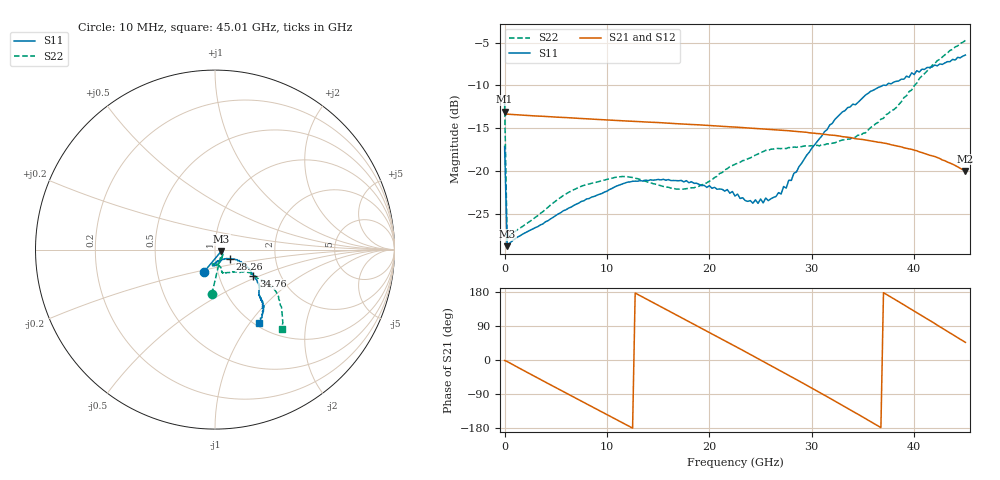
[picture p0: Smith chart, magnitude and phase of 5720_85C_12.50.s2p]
! Device:  ADRF5720
! Description: 0.5dB LSB GaAs MMIC 6-bit Digital Attenuator
! Frequency:  0.000009 -  40 GHz
! Ports:
!	RF1	= Port 1
!	RF2	= Port 2
! Vdd:  3.3 Volt
! Vss:  -3.3 Volt
! Control:  0/3.3 Volt
! State:  12.50 dB attenuation
! Data:  The device was measured using G-S-G Probes on a matrix board.
!  Data was collected using an calibrated 4 port network analyzer.
!  The reference plane for this measurement is at the launchers.
! Note:  Analog Devices supplies this data as a sample of measured data
!  for this product.  Your particular data for this product may vary.
!  Data was taken at 85 degrees C.
!  Analog Devices reserves the right to change this data at anytime.
# GHZ S DB R 45.0
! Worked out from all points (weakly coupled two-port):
!   181 points, 10 MHz to 45.01 GHz, reference 45 ohm
!   highest |S21| = -13.07 dB at 10 MHz (marker M1); lowest = -20.0 dB at 45.01 GHz (marker M2)
!   lowest |S11| = -28.8 dB at 260 MHz (marker M3), VSWR 1.08, Z = 48.3 - j0.813 ohm
!   |S11| at or under -10 dB: start of sweep to 36.96 GHz; 37.1975 GHz to 37.27 GHz (72.5 MHz wide, 0.195 % of centre)
!   |S22| runs from -28.0 to -4.8 dB; largest |S21 - S12| = 0.001
!   S11 on the Smith chart (normalised r, x): 10 MHz: 0.86, -0.22; 28.26 GHz: 1.17, -0.12; 34.76 GHz: 1.46, -0.46; 45.01 GHz: 1.05, -1.11
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0.01  -17.14 -116.3  -13.07 -1.3  -13.05 -1.3  -12.10 -94.1
0.26  -28.81 -13.4  -13.37 -4.0  -13.37 -4.0  -28.03 -12.8
2.26  -27.09 -15.1  -13.52 -33.4  -13.51 -33.3  -26.08 -25.4
4.26  -25.83 -36.9  -13.66 -62.1  -13.64 -62.1  -24.25 -52.7
7.76  -23.50 -59.0  -13.89 -112.1  -13.88 -112.1  -21.70 -78.5
11.51  -21.52 -78.4  -14.14 -165.5  -14.13 -165.4  -20.66 -95.9
15.26  -21.06 -91.3  -14.37 140.9  -14.36 141.0  -21.74 -99.5
19.01  -21.59 -94.5  -14.62 87.1  -14.61 87.3  -21.80 -82.1
22.76  -22.72 -84.2  -14.90 32.9  -14.89 33.1  -19.11 -72.0
24.26  -23.79 -74.9  -15.02 11.1  -15.01 11.3  -18.31 -72.1
25.01  -23.29 -67.4  -15.07 0.1  -15.06 0.3  -17.87 -73.1
25.26  -23.75 -66.1  -15.09 -3.5  -15.07 -3.3  -17.75 -72.5
25.51  -23.18 -61.7  -15.11 -7.2  -15.09 -7.0  -17.60 -73.2
27.01  -22.71 -43.9  -15.23 -29.4  -15.22 -29.1  -17.40 -71.5
28.26  -20.28 -31.4  -15.37 -48.0  -15.36 -47.7  -17.21 -71.5
30.26  -16.99 -26.2  -15.60 -78.0  -15.58 -77.7  -17.17 -68.0
33.01  -13.10 -29.4  -16.00 -120.0  -15.98 -119.8  -16.39 -57.6
34.76  -11.72 -34.3  -16.29 -146.9  -16.27 -146.6  -15.88 -50.2
37.76  -9.82 -40.7  -16.95 165.5  -16.93 165.9  -12.97 -34.7
41.51  -7.90 -49.0  -18.17 104.6  -18.15 104.9  -8.04 -33.9
43.51  -7.23 -51.5  -19.09 71.5  -19.06 71.8  -5.92 -42.5
45.01  -6.46 -58.9  -20.03 46.6  -20.00 46.9  -4.75 -50.0
